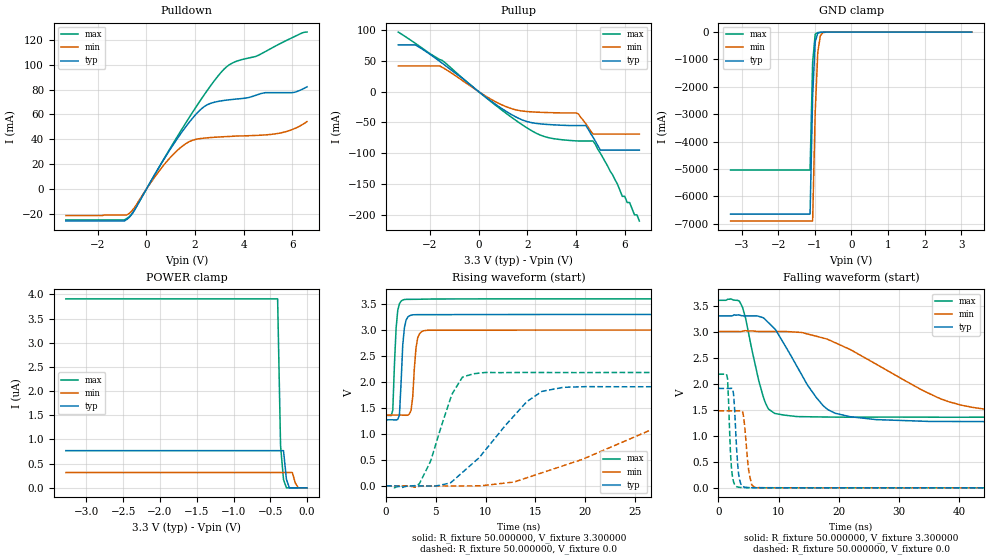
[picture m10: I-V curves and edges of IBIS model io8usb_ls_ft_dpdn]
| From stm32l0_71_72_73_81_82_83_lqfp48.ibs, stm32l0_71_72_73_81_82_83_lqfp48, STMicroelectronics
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|   Model io8usb_ls_ft_dpdn
[Model]  io8usb_ls_ft_dpdn
Model_type I/O
Polarity   Non-Inverting
Enable   Active-Low
Vinl =   0.990000V
Vinh =   2.310000V
Vmeas =  1.650000V
Cref =   50.000000pF
Rref =   100.000000M
Vref =   0.0V
C_comp   4.637700pF   4.580500pF   4.727200pF
[Temperature Range]   25.000000   0.125000k   -40.000000
[Pullup Reference]   3.300000V   3.000000V   3.600000V
[Pulldown Reference]   0.0V   0.0V   0.0V
[POWER Clamp Reference]   3.300000V   3.000000V   3.600000V
[GND Clamp Reference]   0.0V   0.0V   0.0V
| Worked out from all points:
|   slope of the pulldown table from 0 to 0.495 V, typ, clamps not added: 29.7 ohm
|   slope of the pullup table from 0 to 0.495 V, typ, clamps not added: 33.1 ohm
|   GND clamp passes 1 mA (typ) near -0.59 V on its own axis
|   rising waveform, R_fixture 50.000000, V_fixture 3.300000: 20-80 % time 343ps typ, 358ps min, 323ps max; typ from 1.27 V to 3.3 V
|   rising waveform, R_fixture 50.000000, V_fixture 0.0: 20-80 % time 5.3ns typ, 11.9ns min, 2.23ns max; typ from 0 V to 1.91 V
|   falling waveform, R_fixture 50.000000, V_fixture 3.300000: 20-80 % time 6.44ns typ, 15.8ns min, 2.61ns max; typ from 3.3 V to 1.27 V
|   falling waveform, R_fixture 50.000000, V_fixture 0.0: 20-80 % time 573ps typ, 728ps min, 482ps max; typ from 1.91 V to 0 V
[Pulldown]
|Voltage   I(typ)   I(min)   I(max)
-3.3V     -25.41mA   -21mA      -24.52mA
-900mV    -25.41mA   -20.56mA   -24.52mA
-700mV    -22.5mA    -19.36mA   -21.97mA
500mV     16.83mA    13.94mA    16.94mA
1.2V      38.51mA    29.82mA    39.91mA
1.8V      54.63mA    38.53mA    58.7mA
2.4V      66.61mA    41.1mA     76.36mA
3.1V      70.99mA    42.08mA    94.42mA
3.5V      71.99mA    42.47mA    100.9mA
4.5V      75.4mA     43.21mA    106.6mA
5.5V      77.52mA    45.14mA    116.9mA
6.6V      82.21mA    54.31mA    126.1mA
[Pullup]
|Voltage   I(typ)   I(min)   I(max)
-3.3V     75.71mA    41.6mA     96.61mA
-2.6V     75.71mA    41.6mA     78.32mA
-1.6V     49.18mA    41.6mA     52.03mA
800mV     -23.5mA    -18.58mA   -25.36mA
2.2V      -50.59mA   -32.96mA   -64mA
4V        -55.1mA    -34.59mA   -79.98mA
4.4V      -55.1mA    -52mA      -80.18mA
4.7V      -74mA      -69mA      -80.18mA
5V        -95mA      -69mA      -100mA
5.9V      -95mA      -69mA      -170mA
6.2V      -95mA      -69mA      -180mA
6.6V      -95mA      -69mA      -210mA
[GND_clamp]
|Voltage   I(typ)   I(min)   I(max)
-3.3V     -6.648A    -6.902A    -5.041A
-1.13V    -6.648A    -6.902A    -5.041A
-1.06V    -2.348A    -6.902A    -1.115A
-990mV    -354.4mA   -2.925A    -78.01mA
-920mV    -39.6mA    -752.9mA   -17.76mA
-850mV    -11.68mA   -132.4mA   -11.58mA
-780mV    -6.831mA   -24.65mA   -7.717mA
-500mV    -137.7uA   -388.6uA   -81.08uA
3.28V     0A         0A         0A
[POWER_clamp]
|Voltage   I(typ)   I(min)   I(max)
-3.28V    768.6nA    316.4nA    3.906uA
-400mV    768.6nA    316.4nA    3.906uA
-360mV    768.6nA    316.4nA    868nA
-320mV    768.6nA    316.4nA    173.2nA
-280mV    174.9nA    316.4nA    0A
-240mV    0A         316.4nA    0A
-200mV    0A         316.4nA    0A
-160mV    0A         104.7nA    0A
-120mV    0A         0A         0A
0V        0A         0A         0A
[Ramp]
| variable   typ   min   max
dV/dt_r  1.14540/5.29716n   0.88668/11.89056n   1.30955/2.20609n
dV/dt_f  1.21710/6.43294n   0.98220/15.75291n   1.34760/2.61134n
R_load = 50.000000
[Rising Waveform]
R_fixture= 50.000000
V_fixture= 3.300000
V_fixture_min= 3.000000
V_fixture_max= 3.600000
|time   V(typ)   V(min)   V(max)
0s        1.272V     1.363V     1.356V
667.3ps   1.272V     1.363V     1.455V
1.001ns   1.269V     1.363V     3.035V
1.335ns   1.36V      1.363V     3.505V
1.668ns   2.704V     1.362V     3.579V
1.835ns   3.043V     1.36V      3.587V
2.503ns   3.286V     1.451V     3.591V
3.17ns    3.296V     2.845V     3.592V
4.004ns   3.296V     2.993V     3.595V
83.08ns   3.3V       3V         3.6V
[Rising Waveform]
R_fixture= 50.000000
V_fixture= 0.0
V_fixture_min= 0.0
V_fixture_max= 0.0
|time   V(typ)   V(min)   V(max)
0s        5.983uV    5.727uV    14.33uV
3.337ns   -1.076mV   -10.33mV   38.42mV
4.505ns   -2.017mV   -23.88uV   493.7mV
6.673ns   89.86mV    -949.2uV   1.782V
8.842ns   455.1mV    -210.5uV   2.159V
14.18ns   1.625V     156.6mV    2.183V
17.85ns   1.897V     389.5mV    2.181V
31.36ns   1.909V     1.382V     2.181V
36.04ns   1.909V     1.479V     2.182V
83.08ns   1.909V     1.478V     2.181V
[Falling Waveform]
R_fixture= 50.000000
V_fixture= 3.300000
V_fixture_min= 3.000000
V_fixture_max= 3.600000
|time   V(typ)   V(min)   V(max)
0s        3.3V       3V         3.6V
3.837ns   3.305V     3.001V     3.502V
7.341ns   3.268V     3V         1.785V
8.342ns   3.165V     3V         1.508V
9.343ns   3.052V     3V         1.428V
17.35ns   1.581V     2.876V     1.36V
21.86ns   1.365V     2.656V     1.355V
36.2ns    1.274V     1.743V     1.355V
42.38ns   1.272V     1.541V     1.355V
83.08ns   1.272V     1.363V     1.356V
[Falling Waveform]
R_fixture= 50.000000
V_fixture= 0.0
V_fixture_min= 0.0
V_fixture_max= 0.0
|time   V(typ)   V(min)   V(max)
0s        1.909V     1.478V     2.181V
1.502ns   1.908V     1.478V     2.095V
2.002ns   1.908V     1.478V     641.2mV
2.336ns   1.903V     1.478V     198.3mV
3.337ns   264.7mV    1.478V     10.41mV
4.171ns   17.34mV    1.365V     5.458mV
5.005ns   3.12mV     341.3mV    3.462mV
5.506ns   2.474mV    61.42mV    2.128mV
6.34ns    1.954mV    5.931mV    852.3uV
83.08ns   5.983uV    5.727uV    14.33uV
